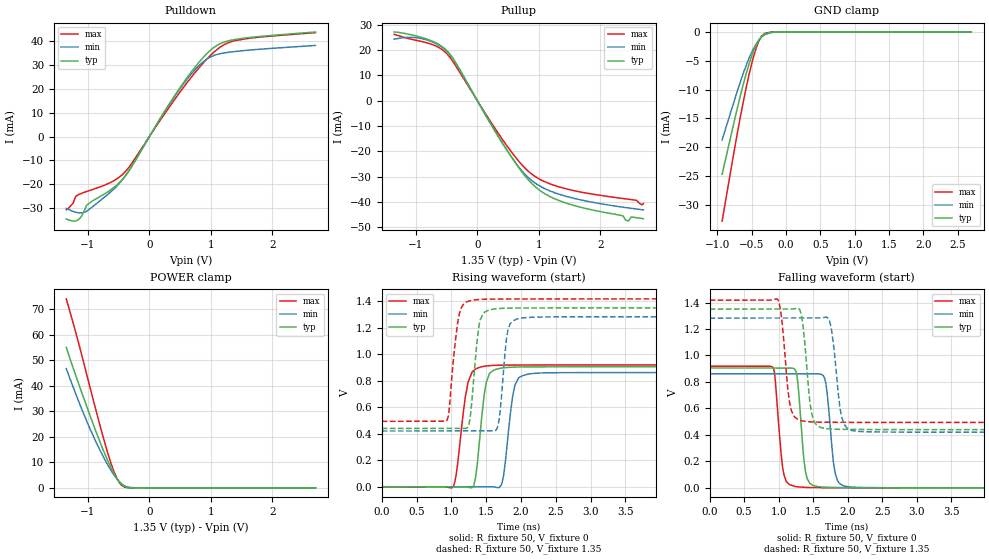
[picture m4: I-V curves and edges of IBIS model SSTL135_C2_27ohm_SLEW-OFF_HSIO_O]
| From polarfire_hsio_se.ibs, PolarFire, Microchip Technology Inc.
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|   Model SSTL135_C2_27ohm_SLEW-OFF_HSIO_O
[Model]   SSTL135_C2_27ohm_SLEW-OFF_HSIO_O
Model_type   Output
Polarity   Non-Inverting
Enable   Active-High
Vmeas =   0.675
Cref =   5p
Rref =   50
Vref =   0.675
|   typ   min   max
C_comp_pullup   1.335e-12   1.335e-12   1.380e-12
C_comp_pulldown  1.335e-12   1.335e-12   1.380e-12
[Temperature Range]  25C   100C   -40C
[Voltage Range]  1.35   1.2825   1.4175
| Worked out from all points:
|   slope of the pulldown table from 0 to 0.203 V, typ, clamps not added: 23.4 ohm
|   slope of the pullup table from 0 to 0.203 V, typ, clamps not added: 23.9 ohm
|   GND clamp passes 1 mA (typ) near -0.37 V on its own axis
|   POWER clamp passes 1 mA (typ) near -0.43 V on its own axis
|   rising waveform, R_fixture 50, V_fixture 0: 20-80 % time 107ps typ, 112ps min, 129ps max; typ from 0 V to 0.906 V
|   rising waveform, R_fixture 50, V_fixture 1.35: 20-80 % time 95ps typ, 85.7ps min, 105ps max; typ from 0.439 V to 1.35 V
|   falling waveform, R_fixture 50, V_fixture 0: 20-80 % time 83.4ps typ, 91.5ps min, 88.1ps max; typ from 0.906 V to 0 V
|   falling waveform, R_fixture 50, V_fixture 1.35: 20-80 % time 95.1ps typ, 105ps min, 95.6ps max; typ from 1.35 V to 0.439 V
[GND Clamp]
| Voltage   I(typ)   I(min)   I(max)
-930.2mV  -24.71mA   -18.73mA   -32.82mA
-708.7mV  -13.23mA   -10.27mA   -17.58mA
-620.2mV  -8.998mA   -7.111mA   -12.02mA
-531.6mV  -5.316mA   -4.365mA   -7.064mA
-487.3mV  -3.767mA   -3.209mA   -4.927mA
-443mV    -2.466mA   -2.228mA   -3.102mA
-398.7mV  -1.449mA   -1.441mA   -1.67mA
-354.4mV  -738.4uA   -854uA     -712.2uA
-310.1mV  -318.4uA   -457.5uA   -228.1uA
-221.5mV  -38.75uA   -96.27uA   -13.59uA
-132.9mV  -3.522uA   -14.87uA   -692.4nA
2.7V      0A         0A         0A
[POWER Clamp]
| Voltage   I(typ)   I(min)   I(max)
-1.35V    55.07mA    46.77mA    74.1mA
-1.196V   44.05mA    36.84mA    60.94mA
-974.5mV  29.03mA    23.74mA    40.36mA
-797.3mV  17.68mA    14.49mA    24.04mA
-664.5mV  10.01mA    8.483mA    12.73mA
-575.9mV  5.63mA     5.093mA    6.421mA
-531.6mV  3.786mA    3.641mA    3.935mA
-487.3mV  2.262mA    2.398mA    2.056mA
-443mV    1.133mA    1.41mA     851.4uA
-354.4mV  127.5uA    344.8uA    50.77uA
-221.5mV  1.715uA    33.09uA    747.7nA
2.7V      0A         0A         0A
[Pullup]
| Voltage   I(typ)   I(min)   I(max)
-1.35V    27.07mA    24.23mA    26.19mA
-885.9mV  24.79mA    24.38mA    23.22mA
-487.3mV  19.51mA    19.27mA    18.34mA
-354.4mV  15.05mA    15.06mA    13.87mA
548.4mV   -22.04mA   -21.98mA   -20.07mA
801.6mV   -30.5mA    -29.75mA   -27.28mA
1.012V    -35.41mA   -33.7mA    -31.03mA
1.571V    -41.44mA   -38.62mA   -35.58mA
2.369V    -45.54mA   -42.11mA   -38.69mA
2.457V    -47.57mA   -42.41mA   -38.97mA
2.502V    -45.96mA   -42.55mA   -39.11mA
2.7V      -46.63mA   -43.19mA   -40.7mA
[Pulldown]
| Voltage   I(typ)   I(min)   I(max)
-1.35V    -34.53mA   -30.07mA   -30.67mA
-1.24V    -35.34mA   -31.31mA   -27.94mA
-1.196V   -35.36mA   -31.68mA   -25.03mA
-1.063V   -31.43mA   -31.77mA   -23.4mA
-1.019V   -28.75mA   -31.25mA   -22.99mA
-531.6mV  -20.35mA   -20.82mA   -17.77mA
-310.1mV  -13.44mA   -13.46mA   -12.09mA
548.4mV   22.34mA    21.88mA    20.4mA
843.8mV   32.26mA    30.64mA    29.92mA
1.055V    37.46mA    34.04mA    35.51mA
1.394V    40.7mA     35.68mA    40.21mA
2.7V      43.82mA    38.2mA     43.57mA
[Ramp]
dV/dt_r   0.543411/0.106968n  0.517156/0.111556n  0.551704/0.129126n
dV/dt_f   0.546308/95.1117p  0.517215/0.104936n  0.554413/95.6175p
R_load = 50
[Rising Waveform]
R_fixture = 50
V_fixture = 0
V_fixture_min = 0
V_fixture_max = 0
| Time   V(typ)   V(min)   V(max)
0s        1.372uV    1.46uV     2.06uV
1.012ns   -674.2uV   -517.5uV   -7.528mV
1.2ns     -799.7uV   -613.9uV   673.6mV
1.321ns   7.099mV    -676uV     875.5mV
1.448ns   579.6mV    -741.1uV   906.8mV
1.549ns   855.2mV    -792.9uV   913.4mV
1.714ns   894.9mV    9.837mV    917.1mV
1.916ns   902.7mV    769.2mV    918.2mV
2.114ns   904.3mV    850.9mV    918.6mV
10ns      905.7mV    861.9mV    919.5mV
[Rising Waveform]
R_fixture = 50
V_fixture = 1.35
V_fixture_min = 1.2825
V_fixture_max = 1.4175
| Time   V(typ)   V(min)   V(max)
0s        439.5mV    420.5mV    493.5mV
936ps     440.2mV    421mV      502.9mV
1.115ns   440.3mV    421mV      1.306V
1.254ns   472.3mV    421.1mV    1.401V
1.303ns   699mV      421.1mV    1.407V
1.455ns   1.305V     421.2mV    1.414V
1.656ns   1.343V     439mV      1.416V
1.81ns    1.347V     1.175V     1.416V
2.011ns   1.348V     1.273V     1.416V
10ns      1.35V      1.282V     1.417V
[Falling Waveform]
R_fixture = 50
V_fixture = 0
V_fixture_min = 0
V_fixture_max = 0
| Time   V(typ)   V(min)   V(max)
0s        905.7mV    861.9mV    919.5mV
917ps     905mV      861.5mV    907.6mV
1.075ns   904.9mV    861.4mV    101.3mV
1.233ns   895.1mV    861.3mV    10.74mV
1.388ns   122.9mV    861.2mV    3.593mV
1.573ns   8.775mV    860.7mV    1.704mV
1.687ns   4.259mV    775.1mV    1.426mV
1.816ns   2.151mV    115.8mV    1.111mV
1.943ns   1.374mV    13.98mV    840.3uV
10ns      2.222uV    2.525uV    3.14uV
[Falling Waveform]
R_fixture = 50
V_fixture = 1.35
V_fixture_min = 1.2825
V_fixture_max = 1.4175
| Time   V(typ)   V(min)   V(max)
0s        1.35V      1.282V     1.417V
986ps     1.351V     1.283V     1.424V
1.054ns   1.351V     1.283V     1.226V
1.154ns   1.351V     1.283V     653.3mV
1.351ns   1.229V     1.283V     504.9mV
1.503ns   513.4mV    1.283V     497.4mV
1.735ns   445.2mV    1.263V     495.6mV
1.91ns    441.9mV    539.5mV    494.9mV
2.063ns   441.2mV    432.9mV    494.6mV
10ns      439.5mV    420.5mV    493.5mV
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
